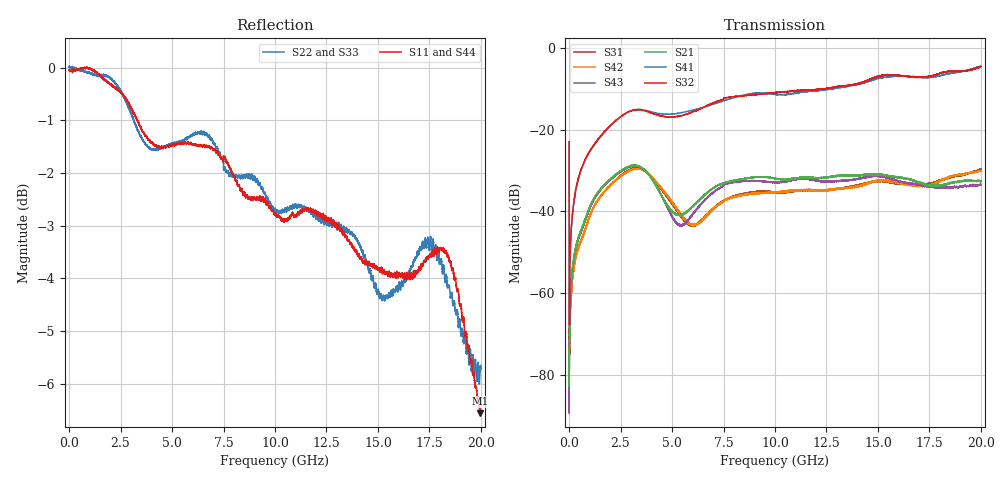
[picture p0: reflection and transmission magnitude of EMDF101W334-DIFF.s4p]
!EMDF101W334
!Johanson Technology Inc.
!www.johansontechnology.com
!Test Board Conditions:
!Substrate Type  RO4350B
!Substrate Thickness  21 mil
!Substrate Dk  3.66
!TL Type: GCPW
!TL Trace Width  40 mil
!TL Gap  17.5 mil
!PART MODE DIFFERENTIAL
!DUT TOPOLOGY	DIFFERENTIAL 4-PORT
# MHz S  dB  R 50
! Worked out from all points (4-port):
!   20001 points, 300 kHz to 20 GHz, reference 50 ohm
!   strongest paths, dB at 300 kHz, 5 GHz, 10 GHz, 15 GHz, 20 GHz:
!     S32: -22.9, -16.8, -10.9, -6.9, -4.5
!     S41: -23.0, -16.1, -11.3, -7.4, -4.4
!     S21: -78.3, -40.0, -31.9, -30.9, -32.6
!     S43: -77.7, -41.3, -32.8, -31.3, -33.4
!     S42: -71.6, -37.6, -35.3, -32.4, -30.0
!     S31: -68.3, -38.1, -35.3, -32.6, -29.6
!   lowest |S11| = -6.6 dB at 19.97 GHz (marker M1), VSWR 2.77, Z = 26.6 - j31.1 ohm
!   |S11| at or under -10 dB: nowhere
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0.3  -0.05 -175.6  -88.59 -137.7  -77.03 -19.1  -22.90 -84.9
     -78.29 57.3  0.03 -175.7  -22.94 -85.3  -72.88 -43.3
     -68.29 -83.6  -22.90 -85.0  -0.05 -175.7  -68.97 -40.9
     -22.98 -84.9  -71.64 46.2  -77.65 39.9  0.07 -175.5
463.293  -0.03 173.8  -46.17 72.5  -48.74 69.9  -31.73 76.8
         -46.09 74.5  -0.03 173.5  -31.61 76.7  -48.70 70.1
         -48.77 69.6  -31.60 76.7  -0.02 173.6  -46.51 73.3
         -31.81 77.1  -49.07 71.5  -46.53 73.0  0.01 173.1
2884.257  -0.67 134.2  -28.97 4.8  -29.90 -2.8  -15.54 26.5
          -28.99 4.9  -0.76 137.0  -15.59 26.0  -30.14 -2.0
          -29.90 -3.1  -15.59 25.8  -0.77 137.5  -29.18 4.8
          -15.54 26.5  -30.17 -2.0  -29.17 4.8  -0.69 136.7
5418.219  -1.44 109.6  -40.89 -32.5  -40.92 -93.0  -15.85 -12.9
          -40.87 -32.5  -1.40 107.4  -16.46 -11.4  -40.71 -93.6
          -41.11 -93.7  -16.53 -11.0  -1.31 108.6  -43.45 -38.9
          -15.82 -13.4  -40.69 -94.2  -43.38 -38.2  -1.57 108.9
12500.11  -2.87 15.6  -31.49 -112.0  -34.80 -152.5  -10.07 -99.8
          -31.59 -112.1  -2.98 16.3  -9.94 -97.8  -34.95 -151.1
          -34.88 -152.2  -9.86 -97.4  -2.85 18.4  -32.49 -112.2
          -10.15 -100.1  -34.87 -151.9  -32.69 -111.6  -2.95 17.7
19967  -6.56 -104.9  -32.94 80.7  -29.67 47.1  -4.72 149.2
       -32.59 79.5  -5.69 -105.8  -4.22 150.8  -29.89 48.6
       -29.68 47.7  -4.50 151.6  -5.81 -97.5  -33.64 85.1
       -4.46 148.5  -30.04 48.8  -33.38 84.2  -6.01 -94.8
20000  -6.51 -106.1  -33.03 78.3  -29.60 46.1  -4.63 148.5
       -32.60 77.7  -5.71 -104.1  -4.25 150.8  -29.92 47.8
       -29.60 46.5  -4.47 151.2  -5.85 -98.0  -33.59 83.2
       -4.39 147.9  -30.04 47.8  -33.36 82.8  -6.07 -95.1
